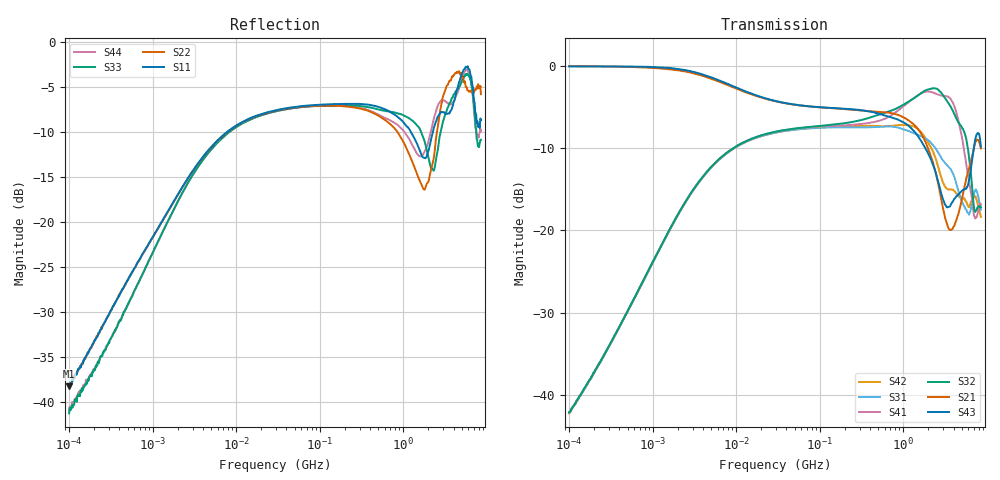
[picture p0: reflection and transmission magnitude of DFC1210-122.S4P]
# Hz S dB R 50
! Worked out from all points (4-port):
!   801 points, 100 kHz to 8.5 GHz, reference 50 ohm
!   strongest paths, dB at 100 kHz, 1.721 MHz, 29.51 MHz, 502.3 MHz, 8.5 GHz:
!     S43: -0.1, -0.3, -4.3, -5.8, -9.8
!     S21: -0.1, -0.5, -4.3, -5.6, -10.0
!     S32: -42.1, -19.3, -8.0, -6.0, -17.2
!     S41: -42.1, -19.3, -8.0, -6.7, -16.9
!     S31: -42.1, -19.3, -8.1, -7.4, -17.5
!     S42: -42.2, -19.4, -8.1, -7.3, -18.3
!   lowest |S11| = -38.2 dB at 100 kHz (marker M1), VSWR 1.02, Z = 50.5 + j1.14 ohm
!   |S11| at or under -10 dB: start of sweep to 7.715 MHz; 1.24 GHz to 2.26 GHz (1.021 GHz wide, 58.3 % of centre)
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100000  -38.24 67.3  -0.06 -0.7  -42.12 -103.1  -42.08 77.0
        -0.06 -0.7  -38.26 68.0  -42.06 77.3  -42.29 -103.9
        -42.09 -102.9  -42.08 76.6  -41.23 64.8  -0.09 -0.5
        -42.10 76.8  -42.20 -103.4  -0.09 -0.5  -40.88 71.9
1.280344e7  -8.70 25.7  -3.20 -13.9  -9.27 -153.2  -9.20 27.9
            -3.21 -13.9  -8.74 25.5  -9.18 28.1  -9.29 -153.0
            -9.28 -153.1  -9.20 28.2  -8.86 27.3  -3.10 -14.5
            -9.21 27.9  -9.30 -153.0  -3.10 -14.5  -8.86 27.4
4.868848e8  -7.15 -4.0  -5.61 -23.3  -7.44 155.1  -6.74 10.5
            -5.61 -23.3  -8.09 -1.9  -6.00 10.7  -7.32 155.8
            -7.45 155.0  -6.02 10.6  -7.45 -6.4  -5.77 -26.3
            -6.76 10.4  -7.33 155.7  -5.77 -26.3  -7.97 -4.8
2.453965e9  -8.87 65.1  -13.04 -127.1  -10.11 59.7  -3.39 -10.3
            -13.02 -127.1  -10.85 16.7  -2.77 -11.5  -11.34 53.3
            -10.08 59.7  -2.78 -11.5  -13.08 62.8  -13.06 -118.5
            -3.40 -10.3  -11.33 53.1  -13.05 -118.5  -7.73 49.9
4.713137e9  -4.34 21.5  -17.48 140.8  -15.70 3.4  -7.24 -50.9
            -17.46 140.3  -3.31 58.0  -7.05 -37.5  -15.94 23.6
            -15.64 3.0  -7.03 -37.6  -4.87 23.1  -15.45 124.3
            -7.24 -51.0  -15.92 23.7  -15.50 124.4  -4.97 25.1
6.946133e9  -6.04 35.4  -10.19 84.6  -15.92 -18.9  -17.77 -46.7
            -10.23 84.6  -5.44 -6.7  -16.82 -54.7  -15.98 -14.3
            -15.91 -19.3  -16.83 -55.4  -6.41 35.7  -10.23 83.2
            -17.82 -46.0  -15.97 -13.8  -10.24 83.7  -6.95 24.8
8.5e9  -8.65 -7.7  -10.05 17.0  -17.46 -135.1  -16.68 -36.5
       -10.04 16.8  -5.78 24.1  -16.99 -35.8  -18.30 -119.9
       -17.47 -134.6  -17.21 -35.9  -10.84 -12.4  -9.93 -1.1
       -16.85 -36.7  -18.34 -117.9  -9.83 -0.9  -9.93 -10.6
